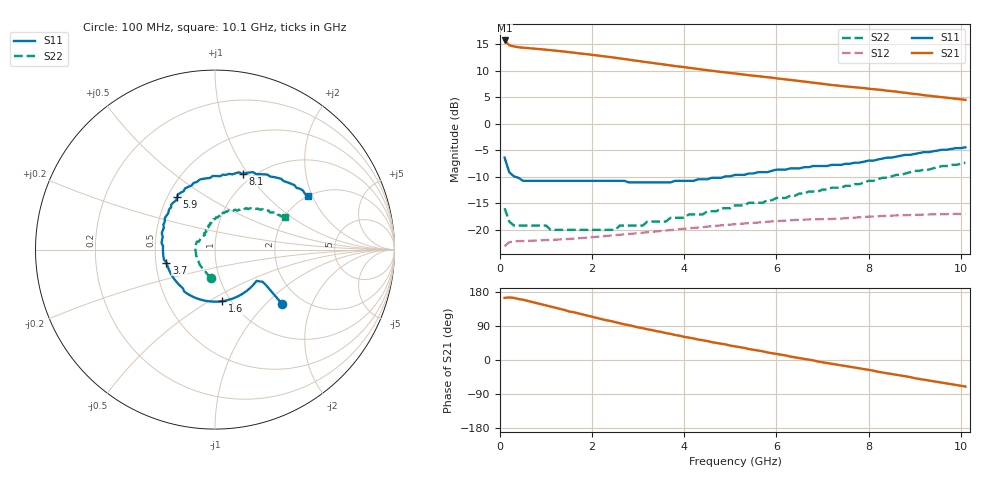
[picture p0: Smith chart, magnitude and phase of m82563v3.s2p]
!	MGA-82563 S PARAMETERS
!	Vd = 3 V LAST UPDATED 3-12-96
# ghz	s ma r	50
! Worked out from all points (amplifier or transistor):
!   101 points, 100 MHz to 10.1 GHz, reference 50 ohm
!   highest |S21| = 15.7 dB at 100 MHz (marker M1)
!   |S21| within 3 dB of that: start of sweep to 2.263 GHz
!   unconditionally stable (mu >= 1): start of sweep to end of sweep
!   at 1.7 GHz: K = 1.36, MAG = 13.8 dB, |S12| = -21.6 dB
!   at 5.1 GHz: K = 1.49, MAG = 10.1 dB, |S12| = -18.9 dB
!   at 10.1 GHz: K = 1.45, MAG = 6.8 dB, |S12| = -17.0 dB
!   lowest NFmin = 2.10 dB at 500 MHz
!   S11 on the Smith chart (normalised r, x): 100 MHz: 1.59, -1.25; 1.6 GHz: 0.91, -0.57; 3.7 GHz: 0.57, -0.09; 5.9 GHz: 0.56, +0.38; 8.1 GHz: 0.89, +0.95; 10.1 GHz: 2.00, +1.87
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0.1  0.48 -39.0  6.1 164.0  0.07026 27.0  0.16 -99.0
0.2  0.35 -35.0  5.5 165.0  0.0764 14.0  0.12 -135.0
0.3  0.32 -34.0  5.36 164.0  0.07772 10.0  0.11 -152.0
1  0.29 -58.0  4.99 144.0  0.08016 3.0  0.11 156.0
1.4  0.29 -74.0  4.79 132.0  0.08178 2.0  0.1 144.0
1.5  0.29 -79.0  4.73 128.0  0.08224 2.0  0.1 142.0
1.6  0.29 -82.0  4.68 126.0  0.08283 2.0  0.1 140.0
1.8  0.29 -90.0  4.57 120.0  0.08404 1.0  0.1 135.0
2.1  0.29 -102.0  4.41 111.0  0.08609 1.0  0.1 130.0
2.5  0.29 -118.0  4.19 100.0  0.08919 -1.0  0.1 124.0
3  0.28 -138.0  3.91 86.0  0.09324 -3.0  0.11 118.0
3.5  0.28 -158.0  3.65 74.0  0.09775 -6.0  0.12 112.0
3.7  0.28 -165.0  3.55 69.0  0.09962 -7.0  0.13 109.0
4.3  0.3 173.0  3.28 54.0  0.1053 -12.0  0.14 103.0
5.1  0.33 148.0  2.98 36.0  0.1132 -19.0  0.17 93.0
5.9  0.36 126.0  2.72 18.0  0.1203 -28.0  0.19 82.0
6.8  0.4 102.0  2.44 -1.0  0.1258 -38.0  0.23 70.0
7.3  0.41 89.0  2.3 -12.0  0.1275 -44.0  0.25 62.0
8.1  0.45 70.0  2.12 -28.0  0.134 -53.0  0.29 51.0
8.5  0.48 61.0  2.03 -37.0  0.1364 -59.0  0.32 45.0
9.1  0.53 49.0  1.89 -50.0  0.1388 -67.0  0.36 37.0
10.1  0.6 30.0  1.68 -70.0  0.1415 -81.0  0.43 25.0
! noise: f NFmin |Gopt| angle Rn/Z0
0.5  2.1  0.15  25  1.2
1.5  2.1  0.14  65  0.29
2.5  2.12  0.15  94  0.25
3.5  2.16  0.14  134  0.21
4.5  2.2  0.17  177  0.18
5.5  2.19  0.23  -152  0.18
6.5  2.28  0.27  -125  0.23
7.5  2.44  0.31  -97  0.34
8.5  2.5  0.38  -72  0.49
10  2.56  0.51  -40  0.87
